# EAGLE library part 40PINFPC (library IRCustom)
OMRON FPC Connector Source : http://www.omron.com/ecb/products/pdf/fpc.pdf XF2M-4015-rev is good for connecting up 'PSP' SHARP LQ043 LCDs
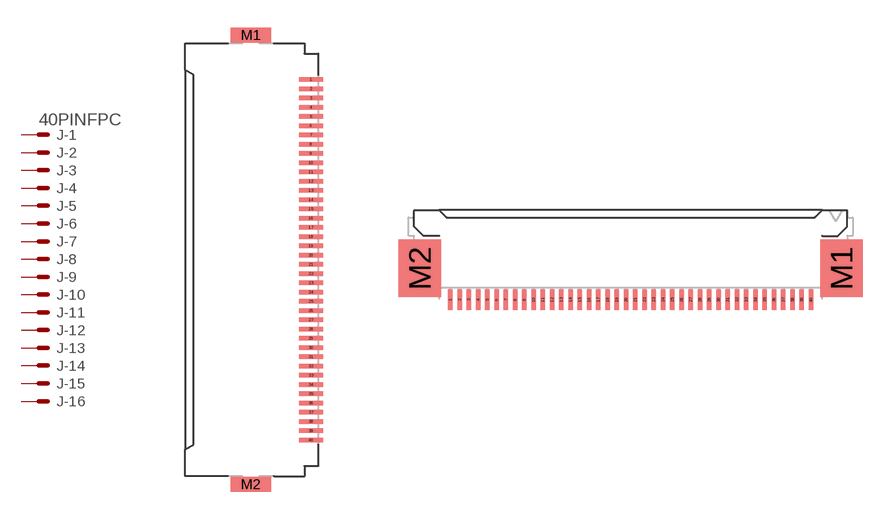
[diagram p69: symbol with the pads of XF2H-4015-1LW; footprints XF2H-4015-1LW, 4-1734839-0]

Designator prefix J; gates -1=PV -2=P -3=P -4=P -5=P -6=P -7=P -8=P -9=P -10=P -11=P -12=P -13=P -14=P -15=P -16=P -17=P -18=P -19=P -20=P -21=P -22=P -23=P -24=P -25=P -26=P -27=P -28=P -29=P -30=P -31=P -32=P -33=P -34=P -35=P -36=P -37=P -38=P -39=P -40=P

## 40PINFPCH15-1LW  [XF2H-4015-1LW]
1  -1:MSV  pas
2  -2:MS  pas
3  -3:MS  pas
4  -4:MS  pas
5  -5:MS  pas
6  -6:MS  pas
7  -7:MS  pas
8  -8:MS  pas
9  -9:MS  pas
10  -10:MS  pas
11  -11:MS  pas
12  -12:MS  pas
13  -13:MS  pas
14  -14:MS  pas
15  -15:MS  pas
16  -16:MS  pas
17  -17:MS  pas
18  -18:MS  pas
19  -19:MS  pas
20  -20:MS  pas
21  -21:MS  pas
22  -22:MS  pas
23  -23:MS  pas
24  -24:MS  pas
25  -25:MS  pas
26  -26:MS  pas
27  -27:MS  pas
28  -28:MS  pas
29  -29:MS  pas
30  -30:MS  pas
31  -31:MS  pas
32  -32:MS  pas
33  -33:MS  pas
34  -34:MS  pas
35  -35:MS  pas
36  -36:MS  pas
37  -37:MS  pas
38  -38:MS  pas
39  -39:MS  pas
40  -40:MS  pas

## 40PINFPCM4-1734839-0  [4-1734839-0]
Pads as for XF2H-4015-1LW

## 40PINFPCR15-4A  [XF2R-4015-4A]
Pads as for XF2H-4015-1LW

## 40PINFPC15-1F-REV  [XF2M-4015-1F-REVERSE]
Pads as for XF2H-4015-1LW

## Footprint XF2H-4015-1LW (pad centres in mm)
Standard Rotary Backlock Type (0.5 mm-pitch) Source : http://www.omron.com/ecb/products/pdf/fpc.pdf
smd 1.3 x 0.25: 1 3.175,9.75; 2 3.175,9.25; 3 3.175,8.75; 4 3.175,8.25; 5 3.175,7.75; 6 3.175,7.25; 7 3.175,6.75; 8 3.175,6.25; 9 3.175,5.75; 10 3.175,5.25; 11 3.175,4.75; 12 3.175,4.25; 13 3.175,3.75; 14 3.175,3.25; 15 3.175,2.75; 16 3.175,2.25; 17 3.175,1.75; 18 3.175,1.25; 19 3.175,0.75; 20 3.175,0.25; 21 3.175,-0.25; 22 3.175,-0.75; 23 3.175,-1.25; 24 3.175,-1.75; 25 3.175,-2.25; 26 3.175,-2.75; 27 3.175,-3.25; 28 3.175,-3.75; 29 3.175,-4.25; 30 3.175,-4.75; 31 3.175,-5.25; 32 3.175,-5.75; 33 3.175,-6.25; 34 3.175,-6.75; 35 3.175,-7.25; 36 3.175,-7.75; 37 3.175,-8.25; 38 3.175,-8.75; 39 3.175,-9.25; 40 3.175,-9.75
smd 2.2 x 0.8: M1 -0.075,12.15; M2 -0.075,-12.15

## Footprint 4-1734839-0 (pad centres in mm)
Reduced-area Rotary Backlock Type (0.5 mm-pitch) Source : http://www.omron.com/ecb/products/pdf/fpc.pdf
smd 0.25 x 1.1: 1 -9.75,-2.54; 2 -9.25,-2.54; 3 -8.75,-2.54; 4 -8.25,-2.54; 5 -7.75,-2.54; 6 -7.25,-2.54; 7 -6.75,-2.54; 8 -6.25,-2.54; 9 -5.75,-2.54; 10 -5.25,-2.54; 11 -4.75,-2.54; 12 -4.25,-2.54; 13 -3.75,-2.54; 14 -3.25,-2.54; 15 -2.75,-2.54; 16 -2.25,-2.54; 17 -1.75,-2.54; 18 -1.25,-2.54; 19 -0.75,-2.54; 20 -0.25,-2.54; 21 0.25,-2.54; 22 0.75,-2.54; 23 1.25,-2.54; 24 1.75,-2.54; 25 2.25,-2.54; 26 2.75,-2.54; 27 3.25,-2.54; 28 3.75,-2.54; 29 4.25,-2.54; 30 4.75,-2.54; 31 5.25,-2.54; 32 5.75,-2.54; 33 6.25,-2.54; 34 6.75,-2.54; 35 7.25,-2.54; 36 7.75,-2.54; 37 8.25,-2.54; 38 8.75,-2.54; 39 9.25,-2.54; 40 9.75,-2.54
smd 2.3 x 3.1: M1 11.4,-0.84; M2 -11.4,-0.84

## Footprint XF2R-4015-4A (pad centres in mm)
Low-profile Rotary Backlock Type (0.5 mm-pitch) Source : http://www.omron.com/ecb/products/pdf/fpc.pdf
smd 0.85 x 0.25: 1 -2.54,9.75; 2 -2.54,9.25; 3 -2.54,8.75; 4 -2.54,8.25; 5 -2.54,7.75; 6 -2.54,7.25; 7 -2.54,6.75; 8 -2.54,6.25; 9 -2.54,5.75; 10 -2.54,5.25; 11 -2.54,4.75; 12 -2.54,4.25; 13 -2.54,3.75; 14 -2.54,3.25; 15 -2.54,2.75; 16 -2.54,2.25; 17 -2.54,1.75; 18 -2.54,1.25; 19 -2.54,0.75; 20 -2.54,0.25; 21 -2.54,-0.25; 22 -2.54,-0.75; 23 -2.54,-1.25; 24 -2.54,-1.75; 25 -2.54,-2.25; 26 -2.54,-2.75; 27 -2.54,-3.25; 28 -2.54,-3.75; 29 -2.54,-4.25; 30 -2.54,-4.75; 31 -2.54,-5.25; 32 -2.54,-5.75; 33 -2.54,-6.25; 34 -2.54,-6.75; 35 -2.54,-7.25; 36 -2.54,-7.75; 37 -2.54,-8.25; 38 -2.54,-8.75; 39 -2.54,-9.25; 40 -2.54,-9.75
smd 1.4 x 1: M1 -0.915,11.05; M2 -0.915,-11.05

## Footprint XF2M-4015-1F-REVERSE (pad centres in mm)
smd 1.1 x 0.25: 1 -2.54,9.75; 2 -2.54,9.25; 3 -2.54,8.75; 4 -2.54,8.25; 5 -2.54,7.75; 6 -2.54,7.25; 7 -2.54,6.75; 8 -2.54,6.25; 9 -2.54,5.75; 10 -2.54,5.25; 11 -2.54,4.75; 12 -2.54,4.25; 13 -2.54,3.75; 14 -2.54,3.25; 15 -2.54,2.75; 16 -2.54,2.25; 17 -2.54,1.75; 18 -2.54,1.25; 19 -2.54,0.75; 20 -2.54,0.25; 21 -2.54,-0.25; 22 -2.54,-0.75; 23 -2.54,-1.25; 24 -2.54,-1.75; 25 -2.54,-2.25; 26 -2.54,-2.75; 27 -2.54,-3.25; 28 -2.54,-3.75; 29 -2.54,-4.25; 30 -2.54,-4.75; 31 -2.54,-5.25; 32 -2.54,-5.75; 33 -2.54,-6.25; 34 -2.54,-6.75; 35 -2.54,-7.25; 36 -2.54,-7.75; 37 -2.54,-8.25; 38 -2.54,-8.75; 39 -2.54,-9.25; 40 -2.54,-9.75
smd 1.5 x 1.7: M1 1.36,11.4; M2 1.36,-11.4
